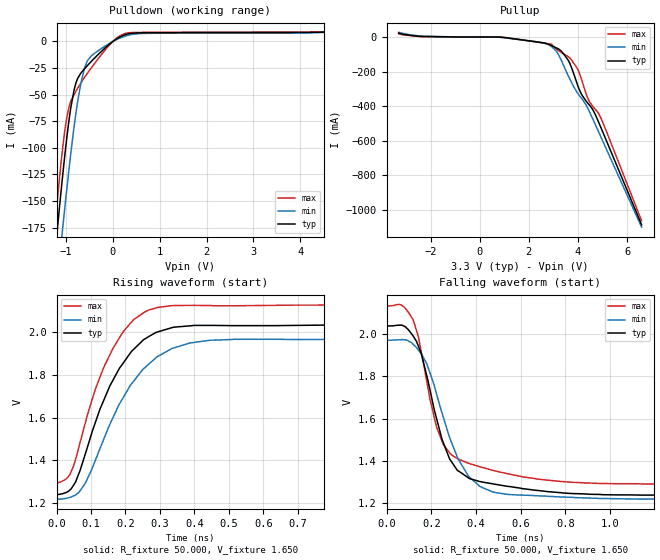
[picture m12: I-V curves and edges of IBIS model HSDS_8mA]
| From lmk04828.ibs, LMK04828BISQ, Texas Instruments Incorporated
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[Model]   HSDS_8mA
Model_type   Output
Polarity   Non-Inverting
Vmeas = 1.9
Vref = 1.9
Cref = 0pF
Rref = 50
|   typ   min   max
|   (nom PVT)   (Fast PVT)   (slow PVT)
C_comp   1.492p   1.392p   1.674p
|C_comp (hi state)   1.492p   1.392p   1.674p
|C_comp (low state)   2.777p   2.419p   2.781p
| Where   nom PVT is  Nominal Process, 3.3V, 27C
|   Fast PVT is Strong Process, 3.45V, -40C
|   Slow PVT is Weak Process, 3.15V, 125C
[Voltage Range]   3.3   3.15   3.45
[Temperature Range]   27   125   -40
[Pullup Reference]   3.3   3.15   3.45
[Pulldown Reference]   0   0   0
[Power Clamp Reference]   3.3   3.15   3.45
[GND Clamp Reference]   0   0   0
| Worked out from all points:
|   slope of the pulldown table from 0 to 0.495 V, typ, clamps not added: 61.7 ohm
|   slope of the pullup table from 0 to 0.495 V, typ, clamps not added: 8 kohm
|   falling waveform, R_fixture 50.000, V_fixture 1.650: 20-80 % time 127ps typ, 150ps min, 119ps max; typ from 2.04 V to 1.24 V
|   rising waveform, R_fixture 50.000, V_fixture 1.650: 20-80 % time 125ps typ, 142ps min, 113ps max; typ from 1.24 V to 2.04 V
[Pulldown]
|   Voltage   I(typ)   I(min)   I(max)
-3.3V     -1.226A    -1.2A      -1.253A
-1.29V    -226.6mA   -272.8mA   -200.2mA
-1.142V   -158.1mA   -207.3mA   -130.7mA
-1.082V   -131.9mA   -181.6mA   -105.5mA
-1.053V   -119.2mA   -168.9mA   -94.06mA
-973.5mV  -87.83mA   -136mA     -69.99mA
-825mV    -45.61mA   -79.95mA   -49.82mA
-686.4mV  -30.15mA   -40.74mA   -39.45mA
-607.2mV  -25.89mA   -25.84mA   -34.12mA
-409.2mV  -16.58mA   -11.85mA   -21.93mA
194.7mV   5.121mA    3.874mA    6.323mA
6.59V     10.59mA    10.66mA    10.59mA
[Pullup]
|   Voltage   I(typ)   I(min)   I(max)
-3.3V     22.42mA    27.3mA     18.86mA
-2.34V    3.185mA    4.961mA    2.641mA
897.6mV   -1.267mA   -2.718mA   -282.3uA
2.363V    -28.99mA   -28.16mA   -29.95mA
2.907V    -48.74mA   -53.27mA   -41.4mA
3.303V    -79.15mA   -129.1mA   -87.94mA
3.679V    -156.2mA   -246.1mA   -122.5mA
3.986V    -278.5mA   -324.2mA   -186mA
4.412V    -384.5mA   -415.9mA   -358.3mA
4.709V    -450mA     -507.1mA   -418.7mA
4.957V    -531.4mA   -585.3mA   -475.6mA
6.59V     -1.086A    -1.1A      -1.063A
[Ramp]
R_load = 50
|   typ   min   max
dV/dt_r   0.471953/1.25144e-10   0.443681/1.42193e-10   0.494567/1.13542e-10
dV/dt_f   0.471995/1.26586e-10   0.443829/1.50046e-10   0.494457/1.19591e-10
[Falling Waveform]
R_fixture = 50.000
V_fixture = 1.650
V_fixture_min = 1.606
V_fixture_max = 1.726
C_fixture = 0.000
|  time   V(typ)   V(min)   V(max)
|   0.000S   2.037V   1.970V   2.131V
|  161.057ps   2.037V   1.970V   2.131V
|  164.182ps   2.037V   1.970V   2.131V
|  171.164ps   2.037V   1.970V   2.131V
|  195.558ps   2.037V   1.971V   2.132V
|  213.447ps   2.038V   1.971V   2.132V
|  216.399ps   2.038V   1.971V   2.132V
|  234.437ps   2.039V   1.971V   2.134V
|  234.563ps   2.039V   1.971V   2.134V
|  239.687ps   2.039V   1.972V   2.135V
|  240.387ps   2.039V   1.972V   2.135V
|  243.475ps   2.039V   1.972V   2.135V
|  253.000ps   2.041V   1.972V   2.138V
|  264.610ps   2.042V   1.973V   2.140V
|  266.721ps   2.042V   1.973V   2.140V
|  271.528ps   2.042V   1.973V   2.140V
|  271.701ps   2.042V   1.973V   2.140V
|  277.139ps   2.043V   1.973V   2.138V
|  280.326ps   2.042V   1.973V   2.136V
|  284.084ps   2.041V   1.974V   2.133V
|  284.198ps   2.041V   1.974V   2.133V
|  291.495ps   2.037V   1.973V   2.127V
|  294.488ps   2.036V   1.973V   2.124V
|  294.993ps   2.035V   1.973V   2.123V
|  297.031ps   2.034V   1.972V   2.121V
|  299.292ps   2.032V   1.972V   2.118V
|  300.474ps   2.030V   1.972V   2.117V
|  307.889ps   2.023V   1.969V   2.106V
|  310.971ps   2.019V   1.967V   2.102V
|  311.265ps   2.019V   1.967V   2.102V
|  325.084ps   2.000V   1.959V   2.078V
|  327.898ps   1.996V   1.956V   2.073V
|  331.337ps   1.991V   1.952V   2.068V
|  344.802ps   1.968V   1.938V   2.022V
|  346.498ps   1.965V   1.936V   2.016V
|  354.512ps   1.944V   1.925V   1.989V
|  367.098ps   1.910V   1.908V   1.919V
|  367.688ps   1.909V   1.907V   1.916V
|  379.107ps   1.859V   1.885V   1.852V
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0s        2.037V     1.97V      2.131V
64.77ps   2.043V     1.973V     2.138V
119ps     1.991V     1.952V     2.068V
180.1ps   1.802V     1.859V     1.774V
223ps     1.603V     1.719V     1.562V
254.2ps   1.485V     1.606V     1.476V
320.8ps   1.352V     1.407V     1.409V
426.9ps   1.3V       1.274V     1.369V
957.6ps   1.241V     1.222V     1.293V
2.788ns   1.238V     1.218V     1.292V
[Rising Waveform]
R_fixture = 50.000
V_fixture = 1.650
V_fixture_min = 1.606
V_fixture_max = 1.726
C_fixture = 0.000
|  time   V(typ)   V(min)   V(max)
|   0.000S   1.238V   1.218V   1.292V
|  164.182ps   1.238V   1.218V   1.292V
|  164.914ps   1.238V   1.218V   1.292V
|  201.430ps   1.239V   1.218V   1.293V
|  221.706ps   1.239V   1.218V   1.293V
|  222.302ps   1.239V   1.218V   1.293V
|  231.199ps   1.239V   1.219V   1.293V
|  234.437ps   1.239V   1.219V   1.293V
|  234.563ps   1.239V   1.219V   1.294V
|  239.687ps   1.240V   1.219V   1.294V
|  240.387ps   1.240V   1.219V   1.295V
|  245.277ps   1.241V   1.219V   1.296V
|  246.344ps   1.241V   1.219V   1.296V
|  249.139ps   1.241V   1.219V   1.297V
|  253.000ps   1.242V   1.219V   1.299V
|  257.642ps   1.244V   1.220V   1.302V
|  259.292ps   1.244V   1.220V   1.304V
|  264.422ps   1.247V   1.221V   1.308V
|  264.610ps   1.247V   1.221V   1.308V
|  266.721ps   1.248V   1.222V   1.310V
|  271.528ps   1.251V   1.223V   1.316V
|  271.701ps   1.251V   1.223V   1.316V
|  273.666ps   1.253V   1.224V   1.320V
|  277.139ps   1.256V   1.225V   1.326V
|  280.326ps   1.261V   1.227V   1.332V
|  284.084ps   1.266V   1.228V   1.346V
|  284.198ps   1.266V   1.228V   1.347V
|  291.495ps   1.284V   1.234V   1.374V
|  294.488ps   1.292V   1.236V   1.389V
|  294.993ps   1.293V   1.236V   1.392V
|  297.031ps   1.298V   1.238V   1.403V
|  299.292ps   1.307V   1.240V   1.416V
|  300.474ps   1.312V   1.242V   1.423V
|  307.889ps   1.343V   1.252V   1.468V
|  310.971ps   1.355V   1.259V   1.487V
|  311.265ps   1.357V   1.260V   1.489V
|  325.084ps   1.428V   1.292V   1.573V
|  327.898ps   1.442V   1.301V   1.590V
|  331.337ps   1.460V   1.313V   1.611V
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0s        1.238V     1.218V     1.292V
38.16ps   1.261V     1.227V     1.332V
54.86ps   1.298V     1.238V     1.403V
112.3ps   1.577V     1.4V       1.733V
163.5ps   1.776V     1.6V       1.925V
224.4ps   1.922V     1.773V     2.061V
292ps     2.002V     1.886V     2.117V
387.5ps   2.031V     1.951V     2.127V
514.2ps   2.032V     1.968V     2.125V
2.758ns   2.037V     1.97V      2.131V
